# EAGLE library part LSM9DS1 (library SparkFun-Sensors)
ST Microelectronics LSM9DS1 9DOF IMU - Accelerometer, Gyroscope & Magnetometer The LSM9DS1 is a versatile, motion-sensing system-in-a-chip. It houses a 3-axis accelerometer, 3-axis gyroscope, and 3-axis magnetometer – nine degrees of freedom (9DOF) in a single IC! The LSM9DS1 is equipped with a digital interface, but even that is flexible: it supports both I2C and SPI, so you’ll be hard-pressed to find a microcontroller it doesn’t work with. Datasheet SparkFun Products SparkFun 9 Degrees of Freedom IMU Breakout - LSM9DS1 (SEN-13284) SparkFun Photon IMU Shield (DEV-13629)
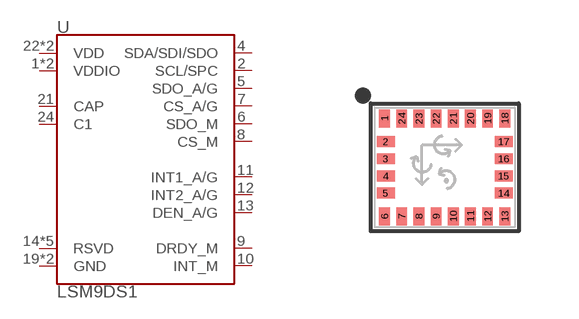
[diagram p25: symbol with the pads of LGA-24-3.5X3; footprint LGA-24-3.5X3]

Designator prefix U

## LSM9DS1 (PROD_ID: IC-12536)  [LGA-24-3.5X3]
1  VDDIO
2  SCL/SPC
3  VDDIO
4  SDA/SDI/SDO
5  SDO_A/G
6  SDO_M
7  CS_A/G
8  CS_M
9  DRDY_M
10  INT_M
11  INT1_A/G
12  INT2_A/G
13  DEN_A/G
14  RSVD
15  RSVD
16  RSVD
17  RSVD
18  RSVD
19  GND
20  GND
21  CAP
22  VDD
23  VDD
24  C1

## Footprint LGA-24-3.5X3 (pad centres in mm)
24-pin LGA (3.5 x 3 mm) Datasheet Specifications: Pin Count: 24 Area: 3.5 x 3.0 mm Pitch: 0.43 mm Devices Using: LSM9DS1
smd 0.27 x 0.45: 1 -1.505,1.225; 6 -1.505,-1.225; 7 -1.075,-1.225; 8 -0.645,-1.225; 9 -0.215,-1.225; 10 0.215,-1.225; 11 0.645,-1.225; 12 1.075,-1.225; 13 1.505,-1.225; 18 1.505,1.225; 19 1.075,1.225; 20 0.645,1.225; 21 0.215,1.225; 22 -0.215,1.225; 23 -0.645,1.225; 24 -1.075,1.225
smd 0.45 x 0.27: 2 -1.475,0.645; 3 -1.475,0.215; 4 -1.475,-0.215; 5 -1.475,-0.645; 14 1.475,-0.645; 15 1.475,-0.215; 16 1.475,0.215; 17 1.475,0.645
